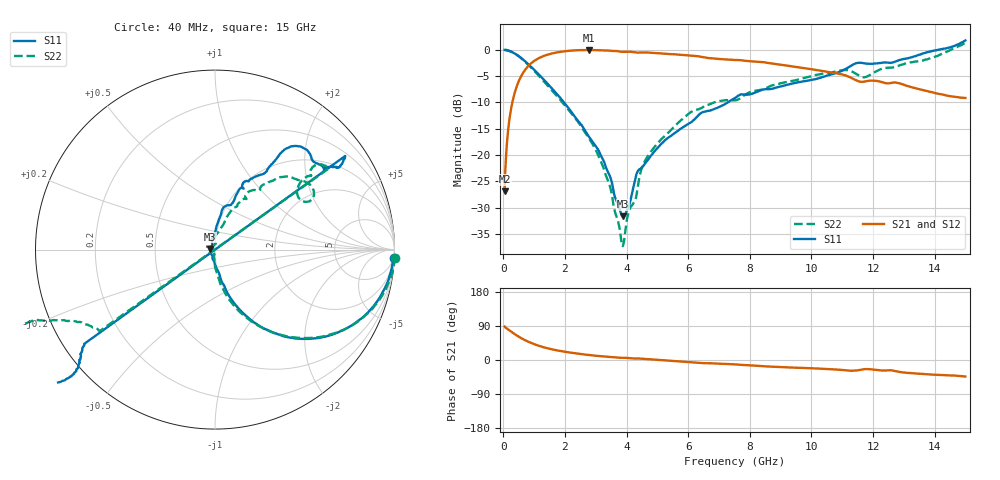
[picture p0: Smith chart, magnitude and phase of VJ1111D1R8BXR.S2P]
! VJ1111D1R8BXR
! DATE 03/08/2022  10:48
! CAPACITORS MOUNTED IN SERIES ON 25 MIL THICK MICROSTRIP SUBSTRATE
# GHz  S  MA  R  50.00
!  FREQ  S11M  S11A  S21M  S21A  S12M  S12A  S22M  S22A
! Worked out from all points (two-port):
!   801 points, 40 MHz to 15 GHz, reference 50 ohm
!   highest |S21| = -0.03 dB at 2.789 GHz (marker M1); lowest = -26.9 dB at 40 MHz (marker M2)
!   |S21| within 3 dB of the highest: 817.8 MHz to 9.245 GHz (8.427 GHz wide, 167 % of centre)
!   lowest |S11| = -31.6 dB at 3.873 GHz (marker M3), VSWR 1.05, Z = 47.5 + j0.275 ohm
!   |S11| at or under -10 dB: 1.969 GHz to 7.29 GHz (5.321 GHz wide, 115 % of centre)
!   |S22| runs from -37.3 to 1.4 dB; largest |S21 - S12| = 0.0068
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0.04  0.9968 -2.6  0.04517 88.4  0.04585 86.6  1.005 -2.5
0.1522  0.9821 -9.4  0.171 80.6  0.1708 80.6  0.9889 -9.6
0.2644  0.9559 -16.3  0.2897 73.9  0.2895 73.8  0.9615 -16.3
0.6384  0.8079 -35.8  0.6033 54.9  0.6024 54.9  0.8036 -35.8
1.4425  0.474 -60.9  0.9011 30.8  0.8989 30.8  0.457 -62.5
2.5458  0.1916 -77.4  0.9919 15.3  0.9888 15.4  0.1824 -81.7
2.7889  0.1479 -79.4  0.9969 13.1  0.9949 13.2  0.1429 -84.0
3.4247  0.06617 -93.8  0.9831 8.2  0.981 8.3  0.05414 -93.8
3.8735  0.02627 173.7  0.956 5.9  0.9532 6.0  0.01361 -173.5
4.341  0.06813 99.6  0.94 3.9  0.9379 4.1  0.04516 96.1
4.528  0.07804 90.0  0.9448 3.2  0.943 3.3  0.07953 87.2
5.0329  0.1191 87.2  0.9274 0.3  0.9241 0.4  0.1313 73.4
6.1175  0.2073 80.2  0.879 -5.8  0.8767 -5.6  0.2592 65.0
7.52  0.3483 68.3  0.8002 -11.5  0.7986 -11.3  0.3309 58.9
10.0258  0.5191 56.7  0.653 -21.8  0.6493 -21.6  0.5641 46.2
11.0543  0.6442 55.8  0.5779 -26.9  0.5761 -26.6  0.6416 33.3
11.5218  0.7526 48.2  0.5031 -27.0  0.5008 -26.8  0.5735 27.6
12.5129  0.7544 36.2  0.4802 -27.1  0.4784 -26.8  0.6746 37.6
13.4105  0.8792 34.9  0.4294 -35.6  0.4278 -35.3  0.7745 36.6
13.5788  0.914 -143.6  0.4172 -36.6  0.4151 -36.2  0.7894 -145.7
14.5138  1.057 -138.7  0.3615 -40.5  0.3613 -40.2  0.9981 -156.6
15  1.227 -141.8  0.3487 -43.7  0.3487 -43.1  1.173 -159.3
